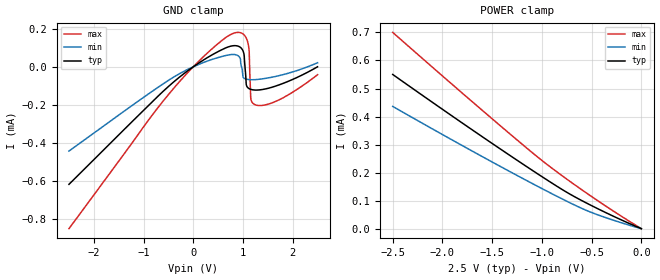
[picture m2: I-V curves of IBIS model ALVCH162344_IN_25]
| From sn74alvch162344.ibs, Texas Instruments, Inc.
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[Model]   ALVCH162344_IN_25
Model_type  Input
Vinl = 0.7
Vinh = 1.7
| variable   typ   min   max
C_comp   2.11pF   1.70pF   2.49pF
[Temperature Range]   40   100   -40
| Ambient temperature   25   85   -40
[Voltage range]   2.5   2.3   2.7
[GND Clamp]
| ALVCH162344_IN_25
|   Voltage   I(typ)   I(min)   I(max)
-2.5V     -616.7uA   -442.1uA   -849.2uA
-505mV    -104.8uA   -72.16uA   -147.6uA
700mV     103.9uA    61.67uA    161.4uA
930mV     104.9uA    50.77uA    179.9uA
995mV     86.34uA    -41.54uA   173.3uA
1.025V    57.1uA     -60.28uA   166.6uA
1.075V    -101.2uA   -65.29uA   145.3uA
1.125V    -114.9uA   -67.29uA   79.22uA
1.16V     -118.7uA   -67.83uA   -170.8uA
1.245V    -122.1uA   -67.4uA    -199.2uA
1.72V     -95.45uA   -46.81uA   -174.1uA
2.5V      6.371pA    21.01uA    -41.71uA
[POWER Clamp]
| ALVCH162344_IN_25
|   Voltage   I(typ)   I(min)   I(max)
-2.5V     550.2uA    436.2uA    700.2uA
-1.6V     328.2uA    257.2uA    422.3uA
-990mV    183.4uA    141.3uA    240.6uA
-740mV    127.8uA    96.19uA    174.3uA
-520mV    85.76uA    60.44uA    119.4uA
-280mV    44.19uA    30.11uA    62.49uA
-31.15fV  6.371pA    6.997pA    6.326pA
